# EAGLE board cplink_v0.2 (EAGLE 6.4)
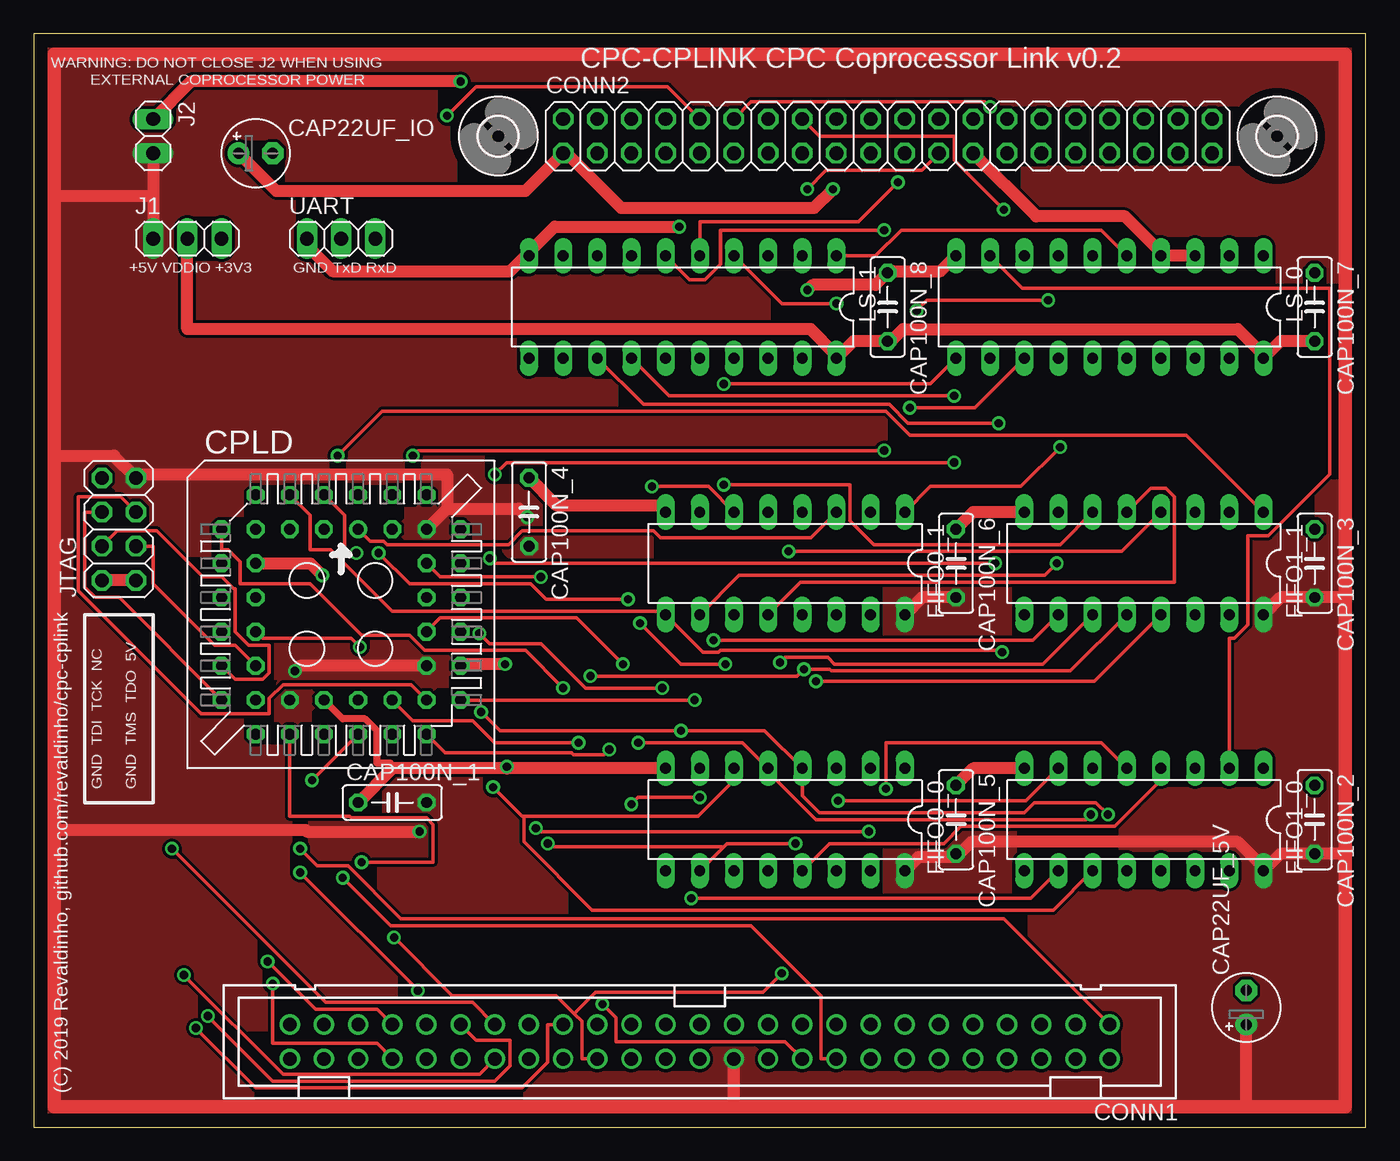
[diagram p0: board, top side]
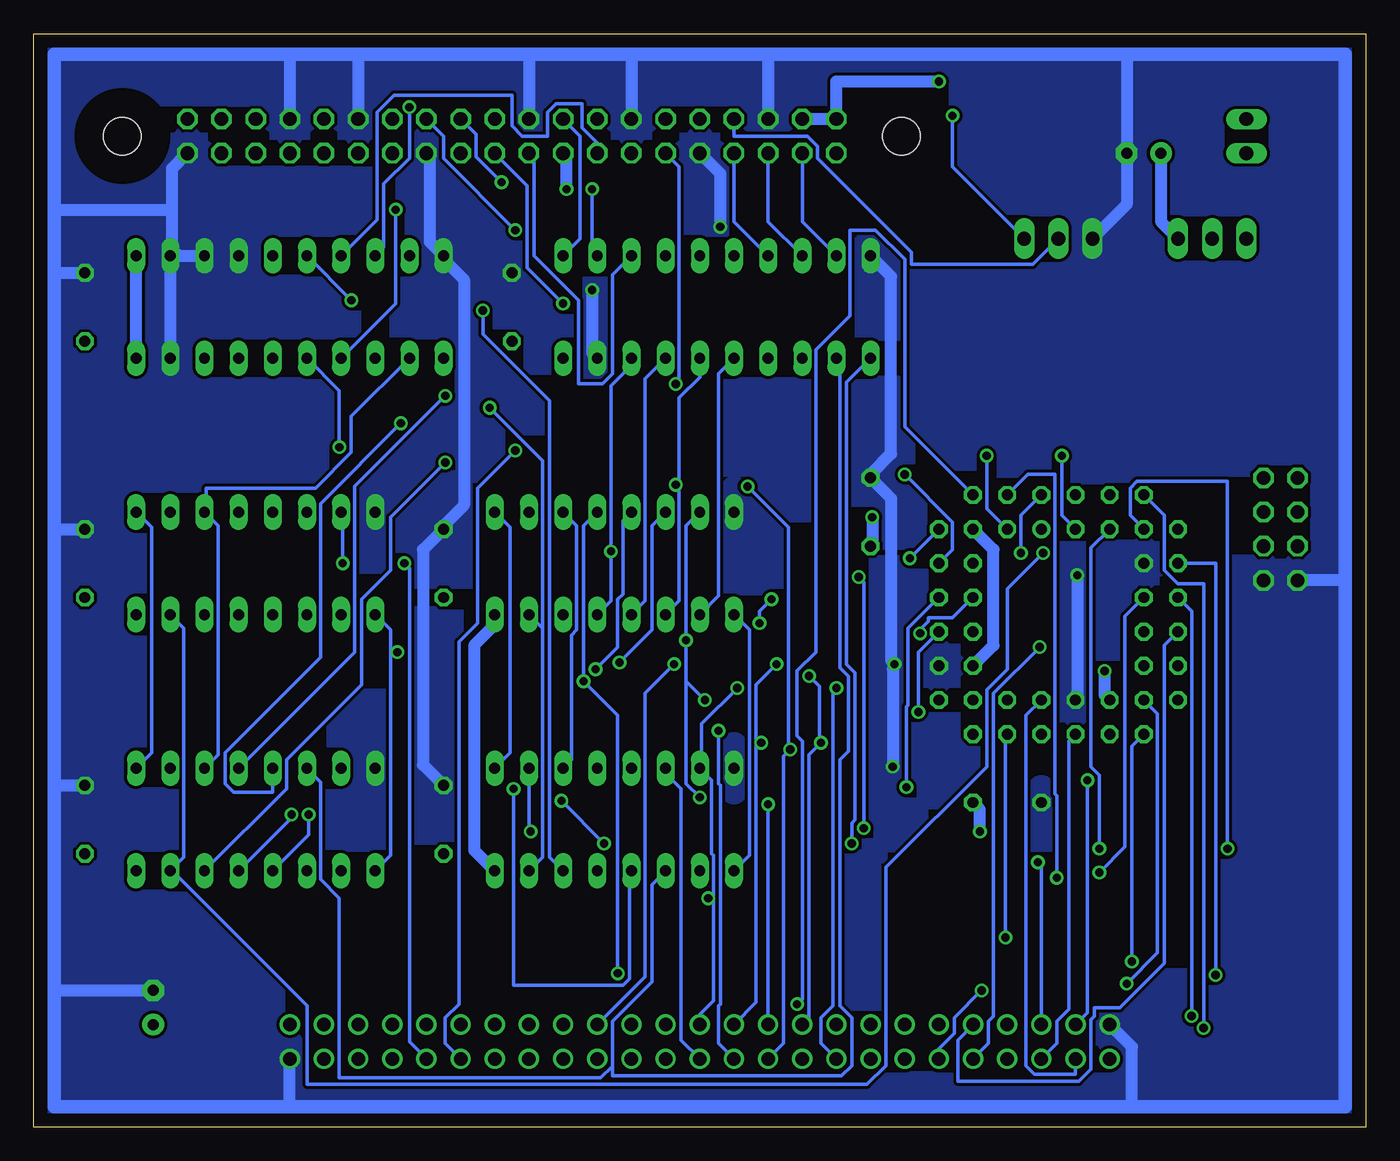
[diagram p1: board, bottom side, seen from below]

Size 99.06 x 81.28 mm. Coordinates in mm from the lower left corner, seen from the top.
Outline: 0,0 99.06,0 99.06,81.28 0,81.28 0,0
Copper layers (1*16): Top 0.035mm / dielectric 1.5mm / Bottom 0.035mm
Design rules "default": minimum track width 10mil, minimum drill 24mil, track to track 8mil, track to pad 8mil, pad to pad 8mil, via to via 8mil, smd to smd 8mil, copper to edge 40mil, drill to drill 8mil, minimum pad ring 10mil, minimum via ring 8mil, stop-mask expansion 4mil, vias tented up to drill 0mil, thermal gap 10mil
Net classes: 0 signal: width 0.254 mm, clearance 0.229 mm; 1 supply: width 0.508 mm, clearance 0.229 mm

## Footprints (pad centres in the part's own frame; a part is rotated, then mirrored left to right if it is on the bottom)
E2,5-5 = drill 0.813 pad 1.6: + -1.27,0 | drill 0.813 pad 1.6 octagon: - 1.27,0
C050-025X075 = drill 0.813 octagon: 1 -2.54,0; 2 2.54,0
PAK100/2500-50 = drill 1 pad 1.422: 1 -30.48,-1.27; 2 -30.48,1.27; 3 -27.94,-1.27; 4 -27.94,1.27; 5 -25.4,-1.27; 6 -25.4,1.27; 7 -22.86,-1.27; 8 -22.86,1.27; 9 -20.32,-1.27; 10 -20.32,1.27; 11 -17.78,-1.27; 12 -17.78,1.27; 13 -15.24,-1.27; 14 -15.24,1.27; 15 -12.7,-1.27; 16 -12.7,1.27; 17 -10.16,-1.27; 18 -10.16,1.27; 19 -7.62,-1.27; 20 -7.62,1.27; 21 -5.08,-1.27; 22 -5.08,1.27; 23 -2.54,-1.27; 24 -2.54,1.27; 25 0,-1.27; 26 0,1.27; 27 2.54,-1.27; 28 2.54,1.27; 29 5.08,-1.27; 30 5.08,1.27; 31 7.62,-1.27; 32 7.62,1.27; 33 10.16,-1.27; 34 10.16,1.27; 35 12.7,-1.27; 36 12.7,1.27; 37 15.24,-1.27; 38 15.24,1.27; 39 17.78,-1.27; 40 17.78,1.27; 41 20.32,-1.27; 42 20.32,1.27; 43 22.86,-1.27; 44 22.86,1.27; 45 25.4,-1.27; 46 25.4,1.27; 47 27.94,-1.27; 48 27.94,1.27; 49 30.48,-1.27; 50 30.48,1.27
2X20 = drill 1.016 octagon: 1 -24.13,-1.27; 2 -24.13,1.27; 3 -21.59,-1.27; 4 -21.59,1.27; 5 -19.05,-1.27; 6 -19.05,1.27; 7 -16.51,-1.27; 8 -16.51,1.27; 9 -13.97,-1.27; 10 -13.97,1.27; 11 -11.43,-1.27; 12 -11.43,1.27; 13 -8.89,-1.27; 14 -8.89,1.27; 15 -6.35,-1.27; 16 -6.35,1.27; 17 -3.81,-1.27; 18 -3.81,1.27; 19 -1.27,-1.27; 20 -1.27,1.27; 21 1.27,-1.27; 22 1.27,1.27; 23 3.81,-1.27; 24 3.81,1.27; 25 6.35,-1.27; 26 6.35,1.27; 27 8.89,-1.27; 28 8.89,1.27; 29 11.43,-1.27; 30 11.43,1.27; 31 13.97,-1.27; 32 13.97,1.27; 33 16.51,-1.27; 34 16.51,1.27; 35 19.05,-1.27; 36 19.05,1.27; 37 21.59,-1.27; 38 21.59,1.27; 39 24.13,-1.27; 40 24.13,1.27
PLCC-S44-SOCKET = drill 0.813: 1 1.27,6.35 | drill 0.813 octagon: 2 -1.27,8.89; 3 -1.27,6.35; 4 -3.81,8.89; 5 -3.81,6.35; 6 -6.35,8.89; 7 -8.89,6.35; 8 -6.35,6.35; 9 -8.89,3.81; 10 -6.35,3.81; 11 -8.89,1.27; 12 -6.35,1.27; 13 -8.89,-1.27; 14 -6.35,-1.27; 15 -8.89,-3.81; 16 -6.35,-3.81; 17 -8.89,-6.35; 18 -6.35,-8.89; 19 -6.35,-6.35; 20 -3.81,-8.89; 21 -3.81,-6.35; 22 -1.27,-8.89; 23 -1.27,-6.35; 24 1.27,-8.89; 25 1.27,-6.35; 26 3.81,-8.89; 27 3.81,-6.35; 28 6.35,-8.89; 29 8.89,-6.35; 30 6.35,-6.35; 31 8.89,-3.81; 32 6.35,-3.81; 33 8.89,-1.27; 34 6.35,-1.27; 35 8.89,1.27; 36 6.35,1.27; 37 8.89,3.81; 38 6.35,3.81; 39 8.89,6.35; 40 6.35,8.89; 41 6.35,6.35; 42 3.81,8.89; 43 3.81,6.35; 44 1.27,8.89
DIL16 = drill 0.813 long: 1 -8.89,-3.81; 2 -6.35,-3.81; 3 -3.81,-3.81; 4 -1.27,-3.81; 5 1.27,-3.81; 6 3.81,-3.81; 7 6.35,-3.81; 8 8.89,-3.81; 9 8.89,3.81; 10 6.35,3.81; 11 3.81,3.81; 12 1.27,3.81; 13 -1.27,3.81; 14 -3.81,3.81; 15 -6.35,3.81; 16 -8.89,3.81
2,8 = hole 2.8: 0,0
1X03 = drill 1.016 long: 1 -2.54,0; 2 0,0; 3 2.54,0
1X02 = drill 1.016 long: 1 -1.27,0; 2 1.27,0
2X04 = drill 1.016 octagon: 1 -3.81,-1.27; 2 -3.81,1.27; 3 -1.27,-1.27; 4 -1.27,1.27; 5 1.27,-1.27; 6 1.27,1.27; 7 3.81,-1.27; 8 3.81,1.27
DIL20 = drill 0.813 long: 1 -11.43,-3.81; 2 -8.89,-3.81; 3 -6.35,-3.81; 4 -3.81,-3.81; 5 -1.27,-3.81; 6 1.27,-3.81; 7 3.81,-3.81; 8 6.35,-3.81; 9 8.89,-3.81; 10 11.43,-3.81; 11 11.43,3.81; 12 8.89,3.81; 13 6.35,3.81; 14 3.81,3.81; 15 1.27,3.81; 16 -1.27,3.81; 17 -3.81,3.81; 18 -6.35,3.81; 19 -8.89,3.81; 20 -11.43,3.81

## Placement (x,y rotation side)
CAP22UF_5V  [E2,5-5]  90.17,8.89 90 top
CAP22UF_IO  [E2,5-5]  16.51,72.39 0 top
CAP100N_1  [C050-025X075]  26.67,24.13 0 top
CAP100N_2  [C050-025X075]  95.25,22.86 270 top
CAP100N_3  [C050-025X075]  95.25,41.91 270 top
CAP100N_4  [C050-025X075]  36.83,45.72 270 top
CAP100N_5  [C050-025X075]  68.58,22.86 270 top
CAP100N_6  [C050-025X075]  68.58,41.91 270 top
CAP100N_7  [C050-025X075]  95.25,60.96 270 top
CAP100N_8  [C050-025X075]  63.5,60.96 270 top
CONN1  [PAK100/2500-50]  49.53,6.35 180 top
CONN2  [2X20]  63.5,73.66 0 top
CPLD  [PLCC-S44-SOCKET]  22.86,38.1 0 top
FIFO0_0  [DIL16]  55.88,22.86 180 top
FIFO0_1  [DIL16]  55.88,41.91 180 top
FIFO1_0  [DIL16]  82.55,22.86 180 top
FIFO1_1  [DIL16]  82.55,41.91 180 top
H1  [2,8]  92.46,73.66 0 top
H2  [2,8]  34.54,73.66 0 top
J1  [1X03]  11.43,66.04 0 top
J2  [1X02]  8.89,73.66 270 top
JTAG  [2X04]  6.35,44.45 90 top
LS_0  [DIL20]  80.01,60.96 180 top
LS_1  [DIL20]  48.26,60.96 180 top
UART  [1X03]  22.86,66.04 0 top

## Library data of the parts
CAP22UF_5V CAP22UF_IO CAP100N_1-CAP100N_8 = resistor
CONN1 = con-3m
CONN2 J1 J2 JTAG UART = pinhead
CPLD FIFO0_0 FIFO0_1 FIFO1_0 FIFO1_1 LS_0 LS_1 = ic-package
H1 H2 = holes

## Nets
A0: CONN1.33 CPLD.6
A1: CONN1.34 CPLD.7
A2: CONN1.35
A3: CONN1.36
A4: CONN1.37 CPLD.8
A5: CONN1.38 CPLD.9
A6: CONN1.39 CPLD.11
A7: CONN1.40 CPLD.12
A8: CONN1.41 CPLD.13
A9: CONN1.42 CPLD.14
A10: CONN1.43 CPLD.18
A11: CONN1.44 CPLD.19
A12: CONN1.45 CPLD.20
A13: CONN1.46 CPLD.22
A14: CONN1.47 CPLD.24
A15: CONN1.48 CPLD.25
BUSACK_B: CONN1.13
BUSRESET_B: CONN1.11
BUSRQ_B: CONN1.14
CLK: CONN1.1 CPLD.5
CURSOR: CONN1.5
D0: CONN1.25 CPLD.36 FIFO0_0.7 FIFO1_0.10
D1: CONN1.26 CPLD.35 FIFO0_0.6 FIFO1_0.11
D2: CONN1.27 CPLD.34 FIFO0_0.5 FIFO1_0.12
D3: CONN1.28 CPLD.33 FIFO0_0.4 FIFO1_0.13
D4: CONN1.29 CPLD.29 FIFO0_1.7 FIFO1_1.10
D5: CONN1.30 CPLD.28 FIFO0_1.6 FIFO1_1.11
D6: CONN1.31 CPLD.27 FIFO0_1.5 FIFO1_1.12
D7: CONN1.32 CPLD.26 FIFO0_1.4 FIFO1_1.13
EXP_B: CONN1.3
FIFO_HOST_DIR: CPLD.38 FIFO0_0.2
FIFO_HOST_DOR: CPLD.37 FIFO1_0.14
FIFO_SLAVE_DIR: FIFO1_0.2 LS_0.9
FIFO_SLAVE_DOR: FIFO0_0.14 LS_0.6
HALT_B: CONN1.17
HOST_FIFO_OEB: CPLD.3 FIFO1_0.1 FIFO1_1.1
HOST_FIFO_RESET: CPLD.4 FIFO0_0.9 FIFO0_1.9 FIFO1_0.9 FIFO1_1.9
HOST_FIFO_SI: CPLD.1 FIFO0_0.3 FIFO0_1.3
HOST_FIFO_SOB: CPLD.2 FIFO1_0.15 FIFO1_1.15
INT_B: CONN1.16
IOREQ_B: CONN1.20 CPLD.40
LPEN: CONN1.4
M1_B: CONN1.22
MREQ_B: CONN1.23
NMI_B: CONN1.15
PI_GPIO_02: CONN2.3 LS_1.9
PI_GPIO_03: CONN2.5 LS_1.8
PI_GPIO_04: CONN2.7 LS_1.7
PI_GPIO_05: CONN2.29
PI_GPIO_06: CONN2.31
PI_GPIO_07: CONN2.26 LS_1.6
PI_GPIO_08: CONN2.24 LS_1.5
PI_GPIO_09: CONN2.21 LS_1.4
PI_GPIO_10: CONN2.19 LS_1.3
PI_GPIO_11: CONN2.23 LS_1.2
PI_GPIO_12: CONN2.32
PI_GPIO_13: CONN2.33
PI_GPIO_14: CONN2.8 UART.2
PI_GPIO_15: CONN2.10 UART.3
PI_GPIO_16: CONN2.36
PI_GPIO_17: CONN2.11 LS_0.11
PI_GPIO_18: CONN2.12 LS_0.8
PI_GPIO_19: CONN2.35
PI_GPIO_20: CONN2.38
PI_GPIO_21: CONN2.40
PI_GPIO_22: CONN2.15 LS_0.7
PI_GPIO_23: CONN2.16 LS_0.14
PI_GPIO_24: CONN2.18 LS_0.5 LS_1.1
PI_GPIO_25: CONN2.22
PI_GPIO_26: CONN2.37
PI_GPIO_27: CONN2.13
RAMDIS: CONN1.6
RAMRD_B: CONN1.7
RD_B: CONN1.19 CPLD.44
READY: CONN1.12 CPLD.43
RESET_B: CONN1.10 CPLD.39
RFSH_B: CONN1.21
ROMDIS: CONN1.8
ROMEN_B: CONN1.9
SCL: CONN2.28
SD0: FIFO0_0.10 FIFO1_0.7 LS_1.11
SD1: FIFO0_0.11 FIFO1_0.6 LS_1.12
SD2: FIFO0_0.12 FIFO1_0.5 LS_1.13
SD3: FIFO0_0.13 FIFO1_0.4 LS_1.14
SD4: FIFO0_1.10 FIFO1_1.7 LS_1.15
SD5: FIFO0_1.11 FIFO1_1.6 LS_1.16
SD6: FIFO0_1.12 FIFO1_1.5 LS_1.17
SD7: FIFO0_1.13 FIFO1_1.4 LS_1.18
SDA: CONN2.27
SLAVE_FIFO_SI: FIFO1_0.3 FIFO1_1.3 LS_0.12
SLAVE_FIFO_SOB: FIFO0_0.15 FIFO0_1.15 LS_0.13
SLAVE_FIFO_WNR: FIFO0_0.1 FIFO0_1.1 LS_0.15
SOUND: CONN1.50
TCK: CPLD.17 JTAG.6
TDI: CPLD.15 JTAG.4
TDO: CPLD.30 JTAG.5
TMS: CPLD.16 JTAG.3
VDD [supply]: CAP22UF_5V.+ CAP100N_1.2 CAP100N_2.2 CAP100N_3.2 CAP100N_4.2 CAP100N_5.2 CAP100N_6.2 CONN1.24 CPLD.21 CPLD.32 CPLD.41 FIFO0_0.16 FIFO0_1.16 FIFO1_0.16 FIFO1_1.16 J1.1 J2.2 JTAG.7
VDD_3V3 [supply]: CAP22UF_IO.+ CONN2.1 CONN2.17 J1.3
VDD_IO [supply]: CAP100N_7.2 CAP100N_8.2 J1.2 LS_0.1 LS_0.20 LS_1.20
VDD_PI [supply]: CONN2.2 CONN2.4 J2.1
VSS [supply]: CAP22UF_5V.- CAP22UF_IO.- CAP100N_1.1 CAP100N_2.1 CAP100N_3.1 CAP100N_4.1 CAP100N_5.1 CAP100N_6.1 CAP100N_7.1 CAP100N_8.1 CONN1.2 CONN1.49 CONN2.6 CONN2.9 CONN2.14 CONN2.20 CONN2.25 CONN2.30 CONN2.34 CONN2.39 CPLD.10 CPLD.23 CPLD.31 FIFO0_0.8 FIFO0_1.8 FIFO1_0.8 FIFO1_1.8 JTAG.1 JTAG.2 LS_0.2 LS_0.3 LS_0.4 LS_0.10 LS_0.19 LS_1.10 LS_1.19 UART.1
WR_B: CONN1.18 CPLD.42

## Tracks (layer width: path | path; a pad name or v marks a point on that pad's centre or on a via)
A0  (via drill 0.61)
  Top 0.254: v12.06,7.37 16.51,2.92 36.32,2.92 38.23,4.83 38.23,7.62 CONN1.33
  Bottom 0.254: CPLD.6 14.99,45.47 14.99,41.4 13.97,40.39 12.06,40.39 v12.06,7.37
A1  (via drill 0.61)
  Top 0.254: CPLD.7 13.97,42.93 14.48,42.93 15.37,42.04 15.37,40.39 20.57,40.39 24.38,36.58 27.94,36.58 29.08,35.43 36.58,35.43 v39.37,32.64
  Bottom 0.254: v39.37,32.64 39.62,32.38 39.62,9.02 40.51,8.13 40.51,6.22 CONN1.34
A4  (via drill 0.61)
  Top 0.254: v10.29,20.7 21.72,9.27 32.64,9.27 CONN1.37
  Bottom 0.254: CPLD.8 17.53,45.47 17.53,47.5 17.02,48.01 10.29,48.01 v10.29,20.7
A5  (via drill 0.61)
  Top 0.254: v11.18,11.3 18.54,3.94 33.15,3.94 CONN1.38
  Bottom 0.254: CPLD.9 11.18,41.91 v11.18,11.3
A6  (via drill 0.61)
  Top 0.254: v12.95,8.26 17.78,3.43 34.29,3.43 35.43,4.57 35.43,6.48 32.89,6.48 CONN1.39
  Bottom 0.254: CPLD.11 12.95,38.35 v12.95,8.26
A7  (via drill 0.61)
  Top 0.254: v28.57,10.16 v19.81,18.92
  Bottom 0.254: CPLD.12 17.91,37.97 17.91,20.83 v19.81,18.92 | v28.57,10.16 30.61,8.13 30.61,6.99 31.75,5.84 CONN1.40
A8
  Bottom 0.254: CPLD.13 14.99,35.81 14.99,12.19 18.29,8.89 20.19,8.89 20.19,8.26 20.45,8 20.45,4.32 21.34,3.43 30.35,3.43 30.35,6.48 CONN1.41
A9  (via drill 0.61)
  Top 0.254: CPLD.14 17.02,36.32 23.62,36.32 v24.26,35.69
  Bottom 0.254: v24.26,35.69 27.69,32.26 27.69,8.26 28.07,7.87 28.07,6.22 CONN1.42
A10  (via drill 0.61)
  Top 0.254: v17.4,12.32 20.95,8.76 25.53,8.76 CONN1.43
  Bottom 0.254: CPLD.18 17.4,28.32 v17.4,12.32
A11  (via drill 0.61)
  Top 0.254: v17.78,10.67 17.78,6.22 25.53,6.22 CONN1.44
  Bottom 0.254: CPLD.19 15.49,30.73 15.49,12.95 v17.78,10.67
A12  (via drill 0.61)
  Top 0.254: CPLD.20 19.05,23.11 23.5,23.11 23.62,22.99 29.21,22.99 29.72,22.48 29.72,19.68 v24.38,19.68
  Bottom 0.254: v24.38,19.68 24.13,19.43 CONN1.45
A13
  Bottom 0.254: CPLD.22 22.1,28.7 22.1,8.76 22.99,7.87 22.99,6.22 CONN1.46
A14  (via drill 0.61)
  Top 0.254: v20.7,25.78 CPLD.24
  Bottom 0.254: v20.7,25.78 20.7,8.51 CONN1.47
A15
  Bottom 0.254: CPLD.25 25.27,30.61 25.27,4.57 24.64,3.94 21.59,3.94 CONN1.48
CLK  (via drill 0.61)
  Top 0.254: v19.81,20.7 21.08,19.43 23.37,19.43 27.3,15.49 72.14,15.49 CONN1.1
  Bottom 0.254: CPLD.5 20.45,43.05 20.45,26.8 19.81,26.16 v19.81,20.7
D0  (via drill 0.61)
  Top 0.254: v33.15,36.7 33.91,35.94 37.72,35.94 41.02,32.64 v46.74,32.64 | FIFO1_0.10 74.17,17.02 v48.9,17.02
  Bottom 0.254: 48.51,17.02 48.51,9.4 49.53,8.38 CONN1.25 | 48.51,17.02 48.51,20.19 48.64,20.32 48.64,25.78 FIFO0_0.7 49.4,26.67 49.4,29.97 v46.74,32.64 | CPLD.36 30.73,37.85 32.51,37.85 32.51,37.59 33.15,36.96 v33.15,36.7 | 48.51,17.02 v48.9,17.02
D1  (via drill 0.61)
  Top 0.254: v34.16,25.27 36.32,23.11 36.45,23.11 | 36.45,23.11 49.4,23.11 52.07,25.78 FIFO0_0.6 | FIFO1_0.11 75.82,16.13 41.53,16.13 36.45,21.21 36.45,23.11
  Bottom 0.254: CPLD.35 34.04,37.08 34.04,31.37 34.16,31.24 v34.16,25.27 | CONN1.26 50.93,6.48 50.93,25.15 52.07,26.29 FIFO0_0.6
D2  (via drill 0.61)
  Top 0.254: CPLD.34 30.23,37.85 40.39,37.85 v43.81,34.42 | v44.96,28.57 52.7,28.57 FIFO0_0.5 54.61,26.42 58.17,22.86 78.23,22.86 v78.61,23.24
  Bottom 0.254: v43.81,34.42 45.34,32.89 45.34,28.57 | 45.34,28.57 45.34,9.27 CONN1.27 | 45.34,28.57 v44.96,28.57 | FIFO1_0.12 78.61,21.72 v78.61,23.24
D3  (via drill 0.61)
  Top 0.254: v33.27,30.86 34.67,29.46 v48.13,29.46 54.36,29.46 FIFO0_0.4 57.15,24.64 58.42,23.37 73.66,23.37 74.42,24.13 78.99,24.13 v79.88,23.24
  Bottom 0.254: CPLD.33 33.27,35.31 v33.27,30.86 | FIFO1_0.13 79.88,22.99 v79.88,23.24 | CONN1.28 48.13,6.22 48.13,9.02 48.01,9.14 48.01,25.4 48.13,25.53 v48.13,29.46
D4  (via drill 0.61)
  Top 0.254: v49.15,31.75 CPLD.29 | FIFO1_1.10 74.3,36.2 v50.55,36.2 | v44.45,24 44.96,24.51 v49.53,24.51
  Bottom 0.254: 50.48,33.08 50.55,33.15 v50.55,36.2 50.55,44.7 FIFO0_1.7 | 50.48,33.08 v49.15,31.75 | v44.45,24 CONN1.29 | v49.53,24.51 50.55,25.53 50.55,33.02 50.48,33.08
D5  (via drill 0.61)
  Top 0.254: CPLD.28 30.61,27.81 40.01,27.81 40.13,27.69 42.42,27.69 v42.8,28.07 | FIFO0_1.6 50.16,47.62 v45.97,47.62 | FIFO1_1.11 75.06,34.42 59.56,34.42 59.05,34.92 55.88,34.92 v55.5,34.54
  Bottom 0.254: CONN1.30 43.31,6.22 43.31,27.56 v42.8,28.07 42.93,28.07 42.93,44.58 v45.97,47.62 | v55.5,34.54 53.09,36.96 53.09,44.7 FIFO0_1.6
D6  (via drill 0.61)
  Top 0.254: FIFO1_1.12 77.09,33.91 59.31,33.91 59.18,34.04 v57.28,34.04 56.77,33.53 v41.4,33.53 | CPLD.27 28.19,30.23 32.64,30.23 34.29,28.57 v40.51,28.57
  Bottom 0.254: FIFO0_1.5 55.24,45.09 55.24,39.62 55.63,39.24 55.63,35.69 v57.28,34.04 | CONN1.31 41.4,8.13 41.4,27.69 v40.51,28.57 40.64,28.57 40.64,32.77 v41.4,33.53
D7  (via drill 0.61)
  Top 0.254: v58.17,33.15 78.87,33.15 FIFO1_1.13 | v26.8,14.1 31.11,9.78 38.86,9.78 40.2,8.45 | 40.2,8.45 40.77,7.87 40.77,5.08 CONN1.32 | v55.63,11.43 54.23,10.03 41.78,10.03 40.2,8.45
  Bottom 0.254: FIFO0_1.4 58.17,44.7 v58.17,33.15 55.63,30.61 v55.63,11.43 | CPLD.26 26.8,29.08 v26.8,14.1
FIFO_HOST_DIR  (via drill 0.61)
  Top 0.254: CPLD.38 30.23,40.89 v37.72,40.89 | v37.34,22.23 37.59,21.97 v62.1,21.97
  Bottom 0.254: v37.72,40.89 37.34,40.51 v37.34,22.23 | v62.1,21.97 62.23,22.1 FIFO0_0.2
FIFO_HOST_DOR  (via drill 0.61)
  Top 0.254: v34.29,48.51 35.18,49.4 v68.45,49.4
  Bottom 0.254: CPLD.37 30.73,42.93 30.73,44.96 v34.29,48.51 | v68.45,49.4 72.52,45.34 72.52,41.4 74.68,39.24 74.68,32.89 80.26,27.3 80.26,25.15 FIFO1_0.14
FIFO_SLAVE_DIR
  Top 0.254: FIFO1_0.2 88.9,36.32 89.28,36.32 90.3,37.34 90.3,43.94 91.82,43.94 96.39,48.51 96.39,62.36 73.53,62.36 LS_0.9
FIFO_SLAVE_DOR  (via drill 0.61)
  Top 0.254: v65.66,60.71 66.42,61.47 v75.44,61.47
  Bottom 0.254: FIFO0_0.14 60.71,20.07 60.71,53.98 65.66,58.93 v65.66,60.71 | LS_0.6 v75.44,61.47
HOST_FIFO_OEB  (via drill 0.61)
  Top 0.254: v22.61,49.91 25.91,53.21 63.37,53.21 65.15,51.44 85.72,51.44 FIFO1_1.1
  Bottom 0.254: CPLD.3 22.61,45.47 v22.61,49.91 | FIFO1_0.1 90.3,27.81 90.3,44.58 FIFO1_1.1
HOST_FIFO_RESET  (via drill 0.61)
  Top 0.254: CPLD.4 20.57,45.47 20.57,42.93 22.1,42.93 26.67,38.35 46.74,38.35 FIFO0_1.9 49.78,35.31 50.93,35.31 51.05,35.43 71.88,35.43 v72.01,35.31
  Bottom 0.254: FIFO1_0.9 72.52,20.19 72.52,35.31 | 72.52,35.31 72.52,36.96 FIFO1_1.9 | FIFO0_0.9 45.85,20.19 45.85,36.96 FIFO0_1.9 | v72.01,35.31 72.52,35.31
HOST_FIFO_SI
  Top 0.254: CPLD.1 25.02,43.56 26.04,43.56 26.29,43.31 35.31,43.31 36.32,44.32 46.1,44.32 46.61,43.81 57.78,43.81 FIFO0_1.3
  Bottom 0.254: FIFO0_0.3 59.05,27.3 59.05,36.58 58.67,36.96 58.67,44.7 FIFO0_1.3
HOST_FIFO_SOB  (via drill 0.61)
  Top 0.254: CPLD.2 23.11,45.47 23.11,42.67 v24,42.67
  Bottom 0.254: FIFO1_1.15 87.88,37.08 87.88,20.07 FIFO1_0.15 88.77,19.05 78.74,9.02 78.74,3.17 37.08,3.17 35.69,4.57 35.69,19.3 28.19,26.8 28.19,32.51 26.67,34.04 26.67,40.01 v24,42.67
IOREQ_B  (via drill 0.61)
  Top 0.254: v42.29,9.14 43.31,8.13 43.31,6.35 55.88,6.35 CONN1.20
  Bottom 0.254: CPLD.40 34.29,52.07 34.29,64.52 36.45,66.67 38.35,66.67 38.35,60.33 40.89,57.78 40.89,35.31 42.29,33.91 42.29,29.08 41.91,28.7 41.91,9.53 v42.29,9.14
PI_GPIO_02
  Bottom 0.254: LS_1.9 41.91,67.31 CONN2.3
PI_GPIO_03
  Bottom 0.254: LS_1.8 44.45,67.31 CONN2.5
PI_GPIO_04
  Bottom 0.254: LS_1.7 46.99,67.31 CONN2.7
PI_GPIO_07  (via drill 0.61)
  Top 0.254: LS_1.6 48.77,62.99 49.91,62.99 51.05,64.14 51.05,66.67 v63.25,66.67
  Bottom 0.254: v63.25,66.67 68.58,72.01 68.58,73.66 CONN2.26
PI_GPIO_08  (via drill 0.61)
  Top 0.254: LS_1.5 49.53,67.31 61.34,67.31 v64.26,70.23
  Bottom 0.254: v64.26,70.23 66.17,72.14 66.17,73.79 CONN2.24
PI_GPIO_09  (via drill 0.61)
  Top 0.254: LS_1.4 55.63,61.21 v59.69,61.21
  Bottom 0.254: v59.69,61.21 62.36,63.88 62.36,69.98 CONN2.21
PI_GPIO_10
  Bottom 0.254: LS_1.3 56.01,63.37 56.01,56.01 56.77,55.24 58.55,55.24 58.55,61.47 61.85,64.77 61.85,72.01 CONN2.19
PI_GPIO_11  (via drill 0.61)
  Top 0.254: v57.53,69.72 58.93,71.12 66.04,71.12 CONN2.23
  Bottom 0.254: LS_1.2 57.53,65.15 v57.53,69.72
PI_GPIO_14
  Bottom 0.254: UART.2 24.77,64.14 33.78,64.14 33.78,65.02 40.77,72.01 40.77,72.9 41.53,73.66 46.99,73.66 CONN2.8
PI_GPIO_15  (via drill 0.61)
  Top 0.254: v30.73,75.18 32.89,77.34 47.12,77.34 CONN2.10
  Bottom 0.254: UART.3 30.73,71.37 v30.73,75.18
PI_GPIO_17  (via drill 0.61)
  Top 0.254: LS_0.11 66.67,55.24 v51.31,55.24
  Bottom 0.254: v51.31,55.24 51.05,55.5 51.05,71.37 CONN2.11
PI_GPIO_18  (via drill 0.61)
  Top 0.254: v71.12,75.82 70.74,76.2 53.34,76.2 CONN2.12
  Bottom 0.254: LS_0.8 73.03,65.41 73.03,70.1 71.12,72.01 v71.12,75.82
PI_GPIO_22
  Bottom 0.254: LS_0.7 73.53,67.44 73.53,75.44 72.26,76.71 63.5,76.71 63.5,74.42 62.74,73.66 60.83,73.66 60.83,75.44 60.2,76.07 58.29,76.07 58.29,74.3 57.15,73.15 CONN2.15
PI_GPIO_23  (via drill 0.61)
  Top 0.254: v72.14,68.2 68.45,71.88 68.45,73.66 58.42,73.66 CONN2.16
  Bottom 0.254: LS_0.14 72.14,61.21 v72.14,68.2
PI_GPIO_24
  Top 0.254: LS_0.5 79.38,66.67 64.52,66.67 62.61,64.77 LS_1.1
  Bottom 0.254: LS_1.1 58.42,66.04 58.42,73.66 CONN2.18
RD_B  (via drill 0.61)
  Top 0.254: v25.65,42.67 27.94,40.39 36.96,40.39 38.1,39.24 v44.2,39.24 | v45.09,37.47 48.13,34.42 v51.44,34.42
  Bottom 0.254: CPLD.44 25.65,45.47 v25.65,42.67 | v44.2,39.24 45.09,38.35 v45.09,37.47 | v51.44,34.42 53.59,32.26 53.59,11.18 CONN1.19
READY  (via drill 0.61)
  Top 0.254: v28.19,49.91 28.57,50.29 v63.25,50.29
  Bottom 0.254: CPLD.43 28.19,45.97 v28.19,49.91 | v63.25,50.29 66.04,47.5 66.04,37.47 67.44,36.07 67.44,9.14 68.45,8.13 68.45,6.22 CONN1.12
RESET_B  (via drill 0.61)
  Top 0.254: v33.91,42.29 34.29,41.91 v71.5,41.91
  Bottom 0.254: v33.91,42.29 CPLD.39 | v71.5,41.91 71.12,41.53 71.12,6.35 CONN1.10
SD0  (via drill 0.61)
  Top 0.254: 51.24,20.77 51.56,21.08 v56.64,21.08 | 51.24,20.77 FIFO0_0.10 | v59.82,24.26 73.79,24.26 FIFO1_0.7 | v38.23,21.08 38.48,20.83 51.18,20.83 51.24,20.77
  Bottom 0.254: v59.82,24.26 v56.64,21.08 | LS_1.11 38.61,55.37 38.61,34.42 37.97,33.78 37.97,22.86 38.23,22.61 v38.23,21.08
SD1
  Bottom 0.254: FIFO0_0.11 53.09,18.03 53.09,10.79 56.01,7.87 56.01,4.57 56.07,4.51 | 56.07,4.51 56.9,3.68 76.33,3.68 76.33,17.02 77.72,18.41 77.72,25.65 FIFO1_0.6 | LS_1.12 39.12,56.9 39.12,34.16 38.48,33.53 38.48,27.94 39.12,27.3 39.12,9.02 38.23,8.13 38.23,4.57 38.99,3.81 56.01,3.81 56.01,4.45 56.07,4.51
SD2  (via drill 0.61)
  Top 0.254: v63.37,25.15 63.37,28.57 79.38,28.57 FIFO1_0.5 | LS_1.13 45.34,53.72 63.63,53.72 65.02,52.32 v71.75,52.32
  Bottom 0.254: FIFO0_0.12 54.74,18.92 54.74,11.05 55.24,10.54 63.37,10.54 v63.37,25.15 | v71.75,52.32 77.72,46.35 77.72,34.92 84.84,27.81 84.84,25.53 84.2,24.89 81.28,24.89 FIFO1_0.5
SD3  (via drill 0.61)
  Top 0.254: FIFO0_0.13 59.18,21.08 67.69,21.08 68.96,22.35 80.39,22.35 83.82,25.78 FIFO1_0.4 | LS_1.14 47.24,54.36 v68.45,54.36
  Bottom 0.254: v68.45,54.36 75.18,47.62 75.18,35.31 FIFO1_0.4
SD4  (via drill 0.61)
  Top 0.254: v76.07,41.91 75.18,41.02 52.45,41.02 FIFO0_1.10
  Bottom 0.254: FIFO0_1.10 48.13,39.5 48.13,56.01 LS_1.15 | FIFO1_1.7 76.07,45.59 v76.07,41.91
SD5  (via drill 0.61)
  Top 0.254: FIFO1_1.6 76.33,43.31 62.48,43.31 60.71,45.09 60.71,47.75 v51.31,47.75
  Bottom 0.254: FIFO0_1.11 51.05,39.12 51.05,47.75 | 51.05,47.75 51.05,54.23 49.53,55.75 LS_1.16 | 51.05,47.75 v51.31,47.75
SD6
  Top 0.254: FIFO1_1.5 83.06,47.5 84.2,47.5 84.84,46.86 84.84,40.51 57.02,40.51 FIFO0_1.12
  Bottom 0.254: FIFO0_1.12 53.59,39.12 53.59,55.63 LS_1.17
SD7  (via drill 0.61)
  Top 0.254: FIFO1_1.4 80.9,42.8 v56.13,42.8
  Bottom 0.254: FIFO0_1.13 56.13,39.12 v56.13,42.8 56.13,55.12 54.61,56.64 LS_1.18
SLAVE_FIFO_SI
  Bottom 0.254: FIFO1_0.3 85.34,27.69 85.34,44.7 FIFO1_1.3 86.23,45.72 86.23,47.5 78.11,47.5 75.44,50.16 75.44,52.83 LS_0.12
SLAVE_FIFO_SOB  (via drill 0.61)
  Top 0.254: LS_0.13 69.98,53.47 v65.15,53.47
  Bottom 0.254: FIFO0_0.15 61.21,20.07 61.21,37.08 61.28,37.15 | FIFO0_1.15 61.28,37.15 | v65.15,53.47 61.21,49.53 61.21,37.21 61.28,37.15
SLAVE_FIFO_WNR  (via drill 0.61)
  Top 0.254: v76.33,50.55 73.41,47.62 66.67,47.62 FIFO0_1.1
  Bottom 0.254: FIFO0_0.1 63.63,27.81 63.63,44.58 FIFO0_1.1 | LS_0.15 76.33,54.74 v76.33,50.55
TCK
  Top 0.254: CPLD.17 6.35,39.37 4.57,39.37 3.81,40.13 3.81,45.72 JTAG.6
TDI
  Top 0.254: CPLD.15 14.99,33.27 17.02,33.27 17.53,33.78 17.53,35.81 16,35.81 14.99,36.83 14.99,40.01 14.86,40.01 13.97,40.89 12.57,40.89 9.14,44.32 6.22,44.32 JTAG.4
TDO
  Top 0.254: CPLD.30 28.07,32.89 18.54,32.89 17.53,31.88 17.53,30.73 12.45,30.73 3.3,39.88 3.3,46.86 6.48,46.86 JTAG.5
TMS
  Top 0.254: CPLD.16 14.99,35.81 13.46,35.81 8.89,40.39 8.89,43.18 JTAG.3
VDD  (via drill 0.61)
  Top 0.889: v19.43,33.91 19.81,34.29 CPLD.32 | v36.7,45.34 36.07,45.97 30.73,45.97 | CPLD.41 30.73,45.97 | FIFO0_0.16 65.79,20.07 68.33,20.07 CAP100N_5.2 68.96,20.45 69.72,21.21 89.53,21.21 91.31,19.43 FIFO1_0.16 92.71,20.32 CAP100N_2.2 97.54,20.32 | FIFO0_1.16 66.04,39.37 CAP100N_6.2 | J2.2 8.89,69.22 | 8.89,69.22 J1.1 | FIFO1_1.16 92.71,39.37 CAP100N_3.2 97.54,39.37 | v28.7,21.97 20.32,21.97 20.19,22.1 1.52,22.1 | 52.07,1.52 CONN1.24 | 1.52,49.91 5.97,49.91 JTAG.7 7.87,48.51 30.73,48.51 30.73,45.97 | 90.17,1.52 CAP22UF_5V.+ | 1.52,69.22 8.89,69.22
  Top 1.016: 1.52,1.52 52.07,1.52 90.17,1.52 97.54,1.52 97.54,20.32 97.54,39.37 97.54,79.76 1.52,79.76 1.52,69.22 1.52,49.91 1.52,22.1 1.52,1.52
  Bottom 0.889: CPLD.21 19.43,32.13 v19.43,33.91 | CPLD.41 27.69,42.93 27.69,35.81 CPLD.32 | CAP100N_4.2 36.7,43.31 v36.7,45.34 | FIFO0_0.16 66.29,20.57 66.29,35.81 64.77,37.34 FIFO0_1.16 | CAP100N_1.2 28.7,23.62 v28.7,21.97
  pour Top: 0,0 0,81.28 99.06,81.28 99.06,0
VDD_3V3  (via drill 0.61)
  Top 0.889: CAP22UF_IO.+ 18.03,69.6 36.58,69.6 CONN2.1 39.75,72.26 43.69,68.33 58.04,68.33 v59.44,69.72
  Bottom 0.889: J1.3 15.24,67.31 CAP22UF_IO.+ | CONN2.17 59.44,72.14 v59.44,69.72
VDD_IO
  Top 0.889: CAP100N_7.2 92.71,58.42 LS_0.20 91.31,57.53 89.53,59.31 64.64,59.31 63.88,58.55 CAP100N_8.2 60.96,58.42 LS_1.20 59.56,57.53 57.78,59.31 11.43,59.31 J1.2
  Bottom 0.889: LS_0.20 LS_0.1
VDD_PI  (via drill 0.61)
  Top 0.889: J2.1 11.68,77.72 v31.75,77.72
  Bottom 0.889: v31.75,77.72 39.37,77.72 CONN2.2 CONN2.4
VSS  (via drill 0.61)
  Top 0.508: CPLD.23 22.99,30.35 24.64,30.35 25.53,29.46 25.53,27.05 26.54,27.05 26.67,26.67
  Top 0.889: v21.46,41.02 20.57,41.91 CPLD.10 | CAP100N_1.1 26.67,26.67 35.18,26.67 | FIFO0_0.8 35.18,26.67 | CPLD.31 31.88,34.42 v35.05,34.42 | FIFO0_1.8 46.48,46.23 38.86,46.23 CAP100N_4.1 | v48.01,66.93 38.73,66.93 36.83,65.02 LS_1.10 36.45,64.64 35.43,63.63 22.23,63.63 20.32,65.53 UART.1 | v35.18,26.8 35.18,26.67 | CAP100N_5.1 69.85,26.67 FIFO1_0.8 | CAP100N_6.1 69.85,45.72 FIFO1_1.8 | v57.53,62.23 57.91,62.61 62.61,62.61 CAP100N_8.1 63.88,63.63 67.44,63.63 LS_0.10 | LS_0.3 LS_0.4 83.69,65.15 81.15,67.69 74.55,67.69 CONN2.25 | JTAG.1 JTAG.2
  Bottom 0.889: CPLD.23 21.46,31.88 v21.46,41.02 | LS_1.10 35.31,63.25 35.31,50.04 36.7,48.64 CAP100N_4.1 35.31,46.74 35.31,34.67 v35.05,34.42 35.18,34.04 v35.18,26.8 | CONN2.9 48.01,70.87 v48.01,66.93 | CAP100N_5.1 70.1,26.92 70.1,42.93 CAP100N_6.1 68.45,44.83 67.06,46.23 67.06,62.99 68.45,64.39 LS_0.10 69.6,65.79 69.6,72.14 CONN2.25 | LS_1.19 57.53,57.53 v57.53,62.23 | LS_0.2 LS_0.19 | CONN2.39 88.77,71.25 88.77,68.2 | 88.77,68.2 88.77,65.15 LS_0.2 | LS_0.3 88.39,64.77 88.39,64.9 LS_0.2 | UART.1 17.78,68.58 CAP22UF_IO.- 17.78,79.76 | 97.54,25.4 CAP100N_2.1 | 97.54,44.45 CAP100N_3.1 | 97.54,63.5 CAP100N_7.1 | 80.01,1.52 CONN1.2 | CONN1.49 17.4,5.97 17.4,1.52 | 44.45,79.76 CONN2.6 | 54.61,79.76 CONN2.14 | 62.23,79.76 CONN2.20 | 74.93,79.76 CONN2.30 | 80.01,79.76 CONN2.34 | 97.54,10.16 CAP22UF_5V.- | 1.52,40.64 JTAG.2 | 97.54,68.2 88.77,68.2
  Bottom 1.016: 1.52,1.52 17.4,1.52 80.01,1.52 97.54,1.52 97.54,10.16 97.54,25.4 97.54,44.45 97.54,63.5 97.54,68.2 97.54,79.76 80.01,79.76 74.93,79.76 62.23,79.76 54.61,79.76 44.45,79.76 17.78,79.76 1.52,79.76 1.52,40.64 1.52,1.52
  pour Bottom: 0,0 0,81.28 99.06,81.28 99.06,0
WR_B  (via drill 0.61)
  Top 0.254: v22.99,18.54 26.54,14.99 53.34,14.99 58.55,9.78 58.55,5.08 CONN1.18
  Bottom 0.254: CPLD.42 25.15,48.51 23.11,48.51 23.11,24.77 22.99,24.64 v22.99,18.54

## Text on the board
tPlace: WARNING: DO NOT CLOSE J2 WHEN USING | CPC-CPLINK CPC Coprocessor Link v0.2 | EXTERNAL COPROCESSOR POWER | +5V VDDIO +3V3 | GND TxD RxD | GND TDI TCK NC | GND TMS TDO 5V | (C) 2019 Revaldinho, github.com/revaldinho/cpc-cplink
